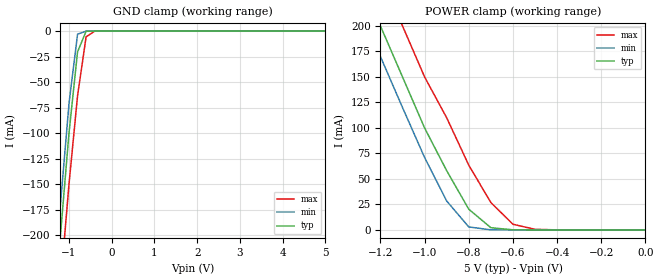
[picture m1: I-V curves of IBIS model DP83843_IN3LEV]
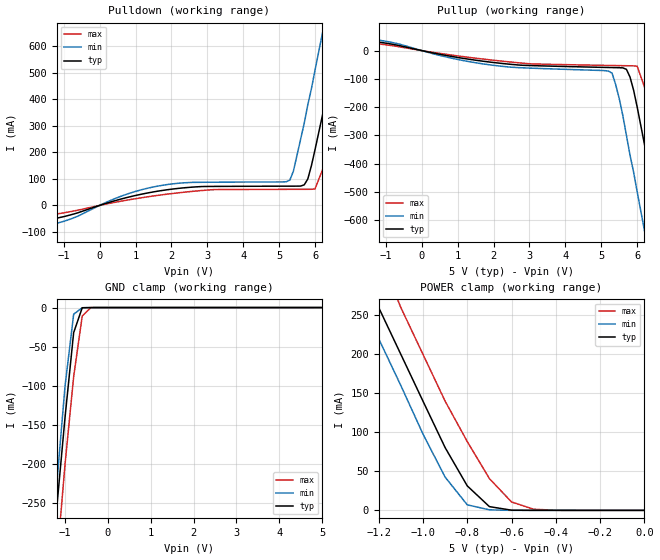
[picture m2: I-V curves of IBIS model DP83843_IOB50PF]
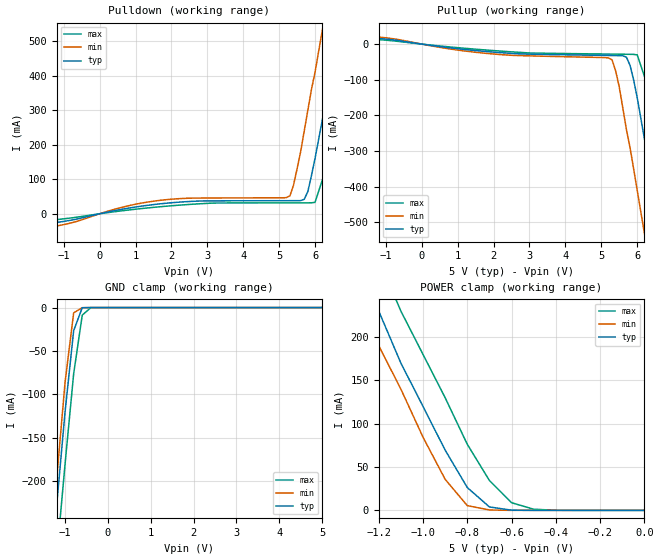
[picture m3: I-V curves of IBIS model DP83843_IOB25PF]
|   National Semiconductor Corporation
|   Local Area Network(LAN) Products Group
|   IBIS Model for DP83843BVJE
|   80L VJE Package
| IBIS file IN3LEV.ibs created by s2ibis2 version 1.1
| North Carolina State University Electronics Research Laboratory  1995
[IBIS ver]   2.1
[File name]   dp83843.ibs
[File Rev]   1.0
[Date]   January 5, 1997
[Source]   Originated at National Semiconductor
[Notes]   From spectre simulated data.
[Disclaimer] Absolutely no guarantees, for modeling purposes only
(C) Copyright National Semiconductor Corporation 1994
   All rights reserved
   National Semiconductor Corporation hereby grants
the user of this IBIS model a non-exclusive, nontransferable
license to use this IBIS model under the following terms.
Before using this IBIS model, the user should read this
license.  If the user does not accept these terms,  the
IBIS model should be returned to National within 30 days.
   The user is granted this license only to use the
IBIS model and is not granted rights to sell, load, rent,
lease or license the IBIS model in whole or in part, or in
modified form to anyone other than user. User may modify
the IBIS model to suit its specific applications but rights
to derivative works and such modifications shall belong to
National.
   This IBIS model is provided on an "AS IS" basis and
National makes absolutely no warranty with respect to the
information contained herein.NATIONAL DISCLAIMS AND CUSTOMER
WAIVES ALL WARRANTIES, EXPRESS OR IMPLIED, INCLUDING
WARRANTIES OF MERCHANTABILITY OR FITNESS FOR A PARTICULAR
PURPOSE. The entire risk as to quality and performance is
with the Customer. ACCORDINGLY, IN NO EVENT SHALL THE
COMPANY BE LIABLE FOR ANY DAMAGES, WHETHER IN CONTRACT OR
TORT,INCLUDING ANY LOST PROFITS OR OTHER INCIDENTAL,
CONSEQUENTIAL, EXEMPLARY, OR PUNITIVE DAMAGES ARISING OUT
OF THE USE OR APPLICATION OF THE IBIS model provided in
this package.Further, National reserves the right to make
changes without notice to any product herein to improve
reliability, function, or design. National does not convey
any license under patent rights or any other intellectual
property rights, including those of third parties.
   National is not obligated to provide maintenance or support
for the licensed IBIS model.
Contact National at ATTN:Signal Management Apps/IBIS MODELS.
2900 Semiconductor Drive, M/S A2595, Santa Clara, CA 95052-8090
|   Component DP83843VJE
[Component]   DP83843BVJE
[Manufacturer]   National Semiconductor Corp.
[Package]
| Note: this data is for the NSC VJE80A package
| variable   typ   min   max
R_pkg   79.00m   50.00m   0.15
L_pkg   3.08nH   2.76nH   3.47nH
C_pkg   0.44pF   0.38pF   0.55pF
[Pin]  signal_name   model_name   R_pin   L_pin   C_pin
1   RESET   DP83843_IOB12PF   79.00m   5.00nH   0.43pF
2   NC   NC   75.00m   4.79nH   0.55pF
3   AN1   DP83843_IN3LEV   71.00m   4.63nH   0.52pF
4   AN0   DP83843_IN3LEV   68.00m   4.55nH   0.48pF
5   SPEED10   DP83843_IOB12PF   67.00m   4.42nH   0.45pF
6   IO_VDD1   POWER   64.00m   4.27nH   0.43pF
7   IO_VSS1   GND   63.00m   4.18nH   0.40pF
8   X2   DP83843_OSC25XO   63.00m   4.08nH   0.39pF
9   X1   DP83843_OSC25XI   62.00m   4.00nH   0.39pF
10   PCS_VDD   POWER   63.00m   3.99nH   0.38pF
11   PCS_VSS   GND   63.00m   3.99nH   0.38pF
12   RXD3   DP83843_IOB50PF   63.00m   4.02nH   0.39pF
13   RXD2   DP83843_IOB50PF   63.00m   4.08nH   0.39pF
14   RXD1   DP83843_IOB50PF   63.00m   4.18nH   0.40pF
15   RXD0   DP83843_IOB50PF   64.00m   4.27nH   0.43pF
16   IO_VDD2   POWER   67.00m   4.42nH   0.45pF
17   IO_VSS2   GND   68.00m   4.55nH   0.48pF
18   RX_CLK   DP83843_IOB50PF   71.00m   4.63nH   0.52pF
19   RX_ER   DP83843_IOB50PF   75.00m   4.79nH   0.55pF
20   RX_DV   DP83843_IOB50PF   79.00m   5.01nH   0.43pF
21   COL   DP83843_IOB50PF   84.00m   5.10nH   0.43pF
22   CRS   DP83843_IOB50PF   78.00m   4.84nH   0.55pF
23   RX_EN   DP83843_IOB12PF   73.00m   4.68nH   0.52pF
24   TX_ER   DP83843_IOB12PF   69.00m   4.57nH   0.48pF
25   TX_EN   DP83843_IOB12PF   67.00m   4.42nH   0.45pF
26   IO_VDD3   POWER   64.00m   4.27nH   0.43pF
27   IO_VSS3   GND   63.00m   4.18nH   0.40pF
28   TXD3   DP83843_IOB12PF   62.00m   4.06nH   0.39pF
29   TXD2   DP83843_IOB12PF   61.00m   3.97nH   0.39pF
30   TXD1   DP83843_IOB12PF   61.00m   3.94nH   0.38pF
31   TXD0   DP83843_IOB12PF   61.00m   3.94nH   0.38pF
32   IO_VSS4   GND   60.00m   3.95nH   0.39pF
33   TX_CLK   DP83843_IOB50PF   60.00m   4.01nH   0.39pF
34   MDIO   DP83843_IOB50PF   61.00m   4.14nH   0.40pF
35   MDC   DP83843_IOB12PF   62.00m   4.22nH   0.43pF
36   IO_VDD5   POWER   63.00m   4.35nH   0.45pF
37   IO_VSS5   GND   66.00m   4.50nH   0.48pF
38   LED_FDPOL   DP83843_IOB12PF   69.00m   4.61nH   0.52pF
39   LED_LINK   DP83843_IOB12PF   74.00m   4.77nH   0.55pF
40   LED_RX   DP83843_IOB12PF   79.00m   5.01nH   0.43pF
41   LED_TX   DP83843_IOB12PF   79.00m   5.01nH   0.43pF
42   LED_COL   DP83843_IOB12PF   73.00m   4.74nH   0.55pF
43   FXTDP   DP83843_PECLIO   71.00m   4.63nH   0.52pF
44   FXTDM   DP83843_PECLIO   69.00m   4.57nH   0.48pF
45   AUIFX_GND   GND   68.00m   4.45nH   0.45pF
46   AUIFX_VDD   POWER   66.00m   4.29nH   0.43pF
47   FXSDP   DP83843_PECLIO   64.00m   4.21nH   0.40pF
48   FXSDM   DP83843_PECLIO   64.00m   4.11nH   0.39pF
49   FXRDM   DP83843_PECLIO   64.00m   4.05nH   0.39pF
50   FXRDP   DP83843_PECLIO   64.00m   4.01nH   0.38pF
51   CP_AGND   GND   64.00m   4.01nH   0.38pF
52   CP_AVDD   POWER   63.00m   4.02nH   0.39pF
53   CPTW_DVSS   GND   62.00m   4.06nH   0.39pF
54   CPTW_DVDD   POWER   62.00m   4.16nH   0.40pF
55   NC   NC   64.00m   4.27nH   0.43pF
56   NC   NC   67.00m   4.42nH   0.45pF
57   ATP_GND   GND   66.00m   4.50nH   0.48pF
58   NC   NC   71.00m   4.63nH   0.52pF
59   NC   NC   75.00m   4.79nH   0.55pF
60   TWREF   DP83843_IOBARE   79.00m   5.01nH   0.43pF
61   BGREF   DP83843_IOBARE   79.00m   5.01nH   0.43pF
62   NC   NC   74.00m   4.77nH   0.55pF
63   THIN   DP83843_IOB25PF   72.00m   4.66nH   0.52pF
64   TW_AGND   GND   69.00m   4.57nH   0.48pF
65   TPRD-   DP83843_IOBARE   63.00m   4.35nH   0.45pF
66   VCM_CAP   DP83843_IOBARE   62.00m   4.22nH   0.43pF
67   TPRD+   DP83843_IOBARE   61.00m   4.14nH   0.40pF
68   TW_AVDD   POWER   63.00m   4.08nH   0.39pF
69   SERIAL10   DP83843_IOB12PF   63.00m   4.02nH   0.39pF
70   SUB_GND   GND   62.00m   3.96nH   0.38pF
71   CD_GND0   GND   62.00m   3.96nH   0.38pF
72   CD_VDD0   POWER   61.00m   3.97nH   0.39pF
73   TPTD-   NC   62.00m   4.06nH   0.39pF
74   TPTD+   NC   63.00m   4.18nH   0.40pF
75   CD_GND1   GND   60.00m   4.17nH   0.43pF
76   CD_VDD1   POWER   61.00m   4.30nH   0.45pF
77   SUB_GND2   GND   69.00m   4.57nH   0.48pF
78   TXAR100   DP83843_IOBARE   74.00m   4.77nH   0.55pF
79   TR_AVDD   POWER   72.00m   4.72nH   0.55pF
80   TR_AGND   GND   78.00m   4.98nH   0.43pF
| Models and submodels in the file (8): DP83843_IN3LEV (Input), DP83843_IOB50PF (I/O), DP83843_IOB25PF (I/O), DP83843_IOB12PF (I/O), DP83843_OSC25XO (I/O), DP83843_OSC25XI (Input), DP83843_PECLIO (I/O), DP83843_IOBARE (Input)
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|   Model IN3LEV
[Model]   DP83843_IN3LEV
Model_type   Input
Vinl =   0.80V
Vinh =   2.00V
Vmeas =   1.50V
C_comp   5.83pF   5.83pF   5.83pF
[Temperature Range]   50.00   -15.00   0.15k
[Voltage Range]   5.00V   4.50V   5.50V
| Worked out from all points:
|   GND clamp passes 1 mA (typ) near -0.61 V on its own axis
|   POWER clamp passes 1 mA (typ) near -0.64 V on its own axis
[GND_clamp]
| voltage   I(typ)   I(min)   I(max)
-5V       -2.2A      -2.18A     -2.25A
-1.4V     -300mA     -270mA     -350mA
-1.2V     -200mA     -170mA     -250mA
-1V       -100mA     -71.1mA    -150mA
-800mV    -20.39mA   -3.02mA    -63.51mA
-600mV    -160uA     -37.59uA   -5.62mA
-400mV    -30.2uA    -33.75uA   -94.45uA
5V        25.89uA    32.55uA    18.68uA
[POWER_clamp]
| voltage   I(typ)   I(min)   I(max)
-5V       2.2A       2.18A      2.25A
-1.3V     250mA      220mA      300mA
-1.2V     200mA      170mA      250mA
-1.1V     150mA      120mA      200mA
-1V       100mA      71.04mA    150mA
-900mV    58.13mA    28.39mA    110mA
-800mV    20.37mA    3mA        63.5mA
-700mV    2.24mA     120uA      26.92mA
-600mV    150uA      34.53uA    5.61mA
-500mV    32.59uA    32.55uA    670uA
0V        25.89uA    32.06uA    18.78uA
|   Model IOB50PF
[Model]   DP83843_IOB50PF
Model_type   I/O
Polarity   Non-Inverting
Enable   Active-High
Vinl =   0.80V
Vinh =   2.00V
Vmeas =   1.50V
Cref =  10.00pF
Rref =  50.00
C_comp   5.83pF   5.83pF   5.83pF
[Temperature Range]   50.00   -15.00   0.15k
[Voltage Range]   5.00V   4.50V   5.50V
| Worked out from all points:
|   slope of the pulldown table from 0 to 0.75 V, typ, clamps not added: 25.6 ohm
|   slope of the pullup table from 0 to 0.75 V, typ, clamps not added: 39.8 ohm
|   GND clamp passes 1 mA (typ) near -0.60 V on its own axis
|   POWER clamp passes 1 mA (typ) near -0.62 V on its own axis
[Pulldown]
| voltage   I(typ)   I(min)   I(max)
-5V       -110mA     -110mA     -110mA
-1.8V     -64.2mA    -86.78mA   -45.05mA
1.9V      59.31mA    78.9mA     42.75mA
5.2V      72.55mA    89.27mA    60.56mA
5.4V      72.62mA    130mA      60.62mA
5.7V      77.51mA    310mA      60.7mA
5.8V      100mA      380mA      60.74mA
6V        210mA      510mA      62.21mA
6.4V      460mA      780mA      200mA
6.8V      730mA      1.05A      450mA
7.2V      1A         1.32A      710mA
10V       2.91A      3.25A      2.59A
[Pullup]
| voltage   I(typ)   I(min)   I(max)
-5V       60.83mA    53.48mA    72.95mA
-1.8V     39.53mA    46.77mA    32.63mA
1.9V      -40.65mA   -50.52mA   -32.72mA
5.2V      -59.76mA   -72.53mA   -52.48mA
5.4V      -60.31mA   -120mA     -52.91mA
5.7V      -66.31mA   -300mA     -53.54mA
5.8V      -93.5mA    -370mA     -53.76mA
6V        -200mA     -500mA     -55.54mA
6.4V      -460mA     -770mA     -200mA
6.8V      -720mA     -1.05A     -450mA
7.2V      -990mA     -1.33A     -710mA
10V       -2.93A     -3.3A      -2.6A
[GND_clamp]
| voltage   I(typ)   I(min)   I(max)
-5V       -2.85A     -2.86A     -2.88A
-1.4V     -390mA     -360mA     -450mA
-1.2V     -260mA     -230mA     -330mA
-1V       -140mA     -100mA     -200mA
-800mV    -32.11mA   -8.53mA    -88.55mA
-600mV    -240uA     -220uA     -10.72mA
-400mV    -410nA     -180nA     -100uA
5V        42.6pA     680nA      -38.59pA
[POWER_clamp]
| voltage   I(typ)   I(min)   I(max)
-5V       2.83A      2.81A      2.87A
-1.3V     330mA      290mA      390mA
-1.2V     260mA      220mA      330mA
-1.1V     200mA      160mA      260mA
-1V       140mA      97.81mA    200mA
-900mV    80.45mA    42.61mA    140mA
-800mV    31.37mA    7.09mA     88.17mA
-700mV    4.78mA     660uA      40.74mA
-600mV    230uA      20.28uA    10.77mA
-500mV    7.54uA     680nA      1.42mA
-400mV    220nA      19.89nA    120uA
0V        42.6pA     31.96pA    2.18nA
[Ramp]
| variable   typ   min   max
dV/dt_r   1.48/1.27n   1.54/0.81n   1.42/1.98n
dV/dt_f   1.82/0.79n   1.92/0.53n   1.65/1.15n
R_load = 50.00
|[Rising Waveform]
|R_fixture = 0.50k
|V_fixture = 0.000
| time   V(typ)   V(min)   V(max)
| Note: If your simulator can handle R_fixture = 0.5k then you
|   can un-comment the Rising and Falling Waveform sections
| 0.000S   -16.65uV   95.93uV   -38.52uV
|  0.40nS   -16.58mV   8.72mV   -2.15mV
|  0.80nS   0.13V   0.85V   -37.01mV
|  1.20nS   1.12V   2.97V   0.14V
|  1.60nS   2.98V   4.07V   0.89V
|  2.00nS   4.14V   4.23V   2.21V
|  2.40nS   4.45V   4.26V   3.47V
|  2.80nS   4.60V   4.26V   4.37V
|  3.20nS   4.64V   4.26V   4.64V
|  3.60nS   4.65V   4.26V   4.80V
|  4.00nS   4.65V   4.26V   4.92V
|  4.40nS   4.65V   4.26V   4.97V
|  4.80nS   4.65V   4.26V   4.98V
|  5.20nS   4.65V   4.26V   4.99V
|  5.60nS   4.65V   4.26V   4.99V
|  6.00nS   4.65V   4.26V   4.99V
|  6.40nS   4.65V   4.26V   4.99V
|  6.80nS   4.65V   4.26V   4.99V
|  7.20nS   4.65V   4.26V   4.99V
|  7.60nS   4.65V   4.26V   4.99V
|  8.00nS   4.65V   4.26V   4.99V
|  8.40nS   4.65V   4.26V   4.99V
|  8.80nS   4.65V   4.26V   4.99V
|  9.20nS   4.65V   4.26V   4.99V
|  9.60nS   4.65V   4.26V   4.99V
| 10.00nS   4.65V   4.26V   4.99V
| 10.40nS   4.65V   4.26V   4.99V
| 10.80nS   4.65V   4.26V   4.99V
| 11.20nS   4.65V   4.26V   4.99V
| 11.60nS   4.65V   4.26V   4.99V
| 12.00nS   4.65V   4.26V   4.99V
| 12.40nS   4.65V   4.26V   4.99V
| 12.80nS   4.65V   4.26V   4.99V
| 13.20nS   4.65V   4.26V   4.99V
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|   Model IOB25PF
[Model]   DP83843_IOB25PF
Model_type   I/O
Polarity   Non-Inverting
Enable   Active-High
Vinl =   0.80V
Vinh =   2.00V
Vmeas =   1.50V
Cref =  10.00pF
Rref =  50.00
C_comp   5.83pF   5.83pF   5.83pF
[Temperature Range]   50.00   -15.00   0.15k
[Voltage Range]   5.00V   4.50V   5.50V
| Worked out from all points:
|   slope of the pulldown table from 0 to 0.75 V, typ, clamps not added: 48.9 ohm
|   slope of the pullup table from 0 to 0.75 V, typ, clamps not added: 74.6 ohm
|   GND clamp passes 1 mA (typ) near -0.61 V on its own axis
|   POWER clamp passes 1 mA (typ) near -0.62 V on its own axis
[Pulldown]
| voltage   I(typ)   I(min)   I(max)
-5V       -56.3mA    -57.5mA    -58.13mA
-1.8V     -33.61mA   -45.47mA   -23.56mA
1.9V      31.02mA    41.31mA    22.34mA
5.2V      37.94mA    46.8mA     31.64mA
5.4V      37.98mA    82.3mA     31.67mA
5.7V      41.97mA    240mA      31.71mA
5.8V      64.43mA    300mA      31.74mA
6V        160mA      410mA      33.06mA
6.4V      380mA      650mA      160mA
6.8V      620mA      890mA      380mA
7.2V      850mA      1.13A      610mA
10V       2.54A      2.83A      2.27A
[Pullup]
| voltage   I(typ)   I(min)   I(max)
-5V       32.51mA    28.61mA    38.95mA
-1.8V     21.13mA    25.02mA    17.42mA
1.9V      -21.7mA    -26.99mA   -17.46mA
5.2V      -31.9mA    -38.79mA   -27.99mA
5.4V      -32.19mA   -75.24mA   -28.22mA
5.7V      -36.74mA   -240mA     -28.56mA
5.8V      -59.45mA   -290mA     -28.68mA
6V        -150mA     -410mA     -30.13mA
6.4V      -380mA     -650mA     -150mA
6.8V      -610mA     -890mA     -370mA
7.2V      -850mA     -1.14A     -600mA
10V       -2.55A     -2.85A     -2.28A
[GND_clamp]
| voltage   I(typ)   I(min)   I(max)
-5V       -2.51A     -2.5A      -2.55A
-1.4V     -350mA     -310mA     -400mA
-1.2V     -230mA     -200mA     -290mA
-1V       -120mA     -85.81mA   -180mA
-800mV    -26.68mA   -6.16mA    -76.31mA
-600mV    -220uA     -110uA     -8.76mA
-400mV    -290nA     -90.39nA   -99.61uA
5V        38.96pA    360nA      -220pA
[POWER_clamp]
| voltage   I(typ)   I(min)   I(max)
-5V       2.5A       2.48A      2.54A
-1.3V     290mA      250mA      340mA
-1.2V     230mA      190mA      290mA
-1.1V     170mA      140mA      230mA
-1V       120mA      84.49mA    180mA
-900mV    69.55mA    35.87mA    130mA
-800mV    26.38mA    5.46mA     76.26mA
-700mV    3.94mA     420uA      34.49mA
-600mV    230uA      11.7uA     8.85mA
-500mV    7.42uA     360nA      1.3mA
-400mV    210nA      10.49nA    120uA
0V        38.96pA    31.74pA    1.99nA
[Ramp]
| variable   typ   min   max
dV/dt_r   0.88/1.00n   0.98/0.67n   0.80/1.49n
dV/dt_f   1.12/0.67n   1.33/0.47n   0.94/0.93n
R_load = 50.00
|[Rising Waveform]
|R_fixture = 0.50k
|V_fixture = 0.000
| Note: If your simulator can handle R_fixture = 0.5k then you
|   can un-comment the Rising and Falling Waveform sections
| time   V(typ)   V(min)   V(max)
|  0.000S   -18.90uV   85.04uV   -34.31uV
|   0.40nS   -21.69mV   35.53mV   -1.96mV
|   0.80nS   0.17V   0.76V   -32.40mV
|   1.20nS   0.99V   2.78V   0.22V
|   1.60nS   2.88V   3.91V   0.90V
|   2.00nS   3.68V   4.05V   1.99V
|   2.40nS   4.25V   4.06V   3.23V
|   2.80nS   4.34V   4.06V   3.88V
|   3.20nS   4.36V   4.06V   4.35V
|   3.60nS   4.36V   4.06V   4.52V
|   4.00nS   4.36V   4.06V   4.57V
|   4.40nS   4.36V   4.06V   4.59V
|   4.80nS   4.36V   4.06V   4.59V
|   5.20nS   4.36V   4.06V   4.59V
|   5.60nS   4.36V   4.06V   4.59V
|   6.00nS   4.36V   4.06V   4.59V
|   6.40nS   4.36V   4.06V   4.59V
|   6.80nS   4.36V   4.06V   4.59V
|   7.20nS   4.36V   4.06V   4.59V
|   7.60nS   4.36V   4.06V   4.59V
|   8.00nS   4.36V   4.06V   4.59V
|   8.40nS   4.36V   4.06V   4.59V
|   8.80nS   4.36V   4.06V   4.59V
|   9.20nS   4.36V   4.06V   4.59V
|   9.60nS   4.36V   4.06V   4.59V
|  10.00nS   4.36V   4.06V   4.59V
|  10.40nS   4.36V   4.06V   4.59V
|  10.80nS   4.36V   4.06V   4.59V
|  11.20nS   4.36V   4.06V   4.59V
|  11.60nS   4.36V   4.06V   4.59V
|  12.00nS   4.36V   4.06V   4.59V
|  12.40nS   4.36V   4.06V   4.59V
|  12.80nS   4.36V   4.06V   4.59V
|  13.20nS   4.36V   4.06V   4.59V
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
